(* Logix 5000 AddOnInstructionDefinition export Banner_K50Z_PD_v4; software revision 33.00 *)

TYPE Banner_K50Z_PD0_v4 :   // Process Data 0 for a K50Z.
STRUCT
   C1_Output_State : SINT;   // 0 = Inactive, 1 = Active
   C2_Output_State : SINT;   // 0 = Inactive, 1 = Active
   Stability_Z1 : SINT;   // 0 = No target or Marginal, 1 = Stable
   Stability_Z2 : SINT;   // 0 = No target or Marginal, 1 = Stable
   Measurement_1 : DINT;   // Default setting is Measurement Value for Zone 1. See IODD for all options.
   Measurement_2 : DINT;   // Default setting is Measurement Value for Zone 2. See IODD for all options.
END_STRUCT
END_TYPE

TYPE Banner_K50Z_PD1_v4 :   // Process Data 1 for a K50Z.
STRUCT
   Measurement_1 : DINT;   // Default setting is Measurement Value for Zone 1. See IODD for all options.
   Measurement_2 : DINT;   // Default setting is Measurement Value for Zone 2. See IODD for all options.
END_STRUCT
END_TYPE

TYPE Banner_K50Z_PD2_v4 :   // Process Data 2 for a K50Z.
STRUCT
   Measurement : DINT;   // Measurement Value
   Measure_Scale : DINT;   // Scale Factor for Measurement
   Stability : SINT;   // 0 = Inactive 1 = Active
   Channel_1 : SINT;   // 0 = Inactive 1 = Active
   Channel_2 : INT;   // 0 = Inactive 1 = Active
END_STRUCT
END_TYPE

TYPE Banner_K50Z_PDIO_v4 :   // Process Data for a K50Z.
STRUCT
   PDI_0 : Banner_K50Z_PD0_v4;   // Input Procoess Data for Configuration 0
   PDI_1 : Banner_K50Z_PD1_v4;   // Input Procoess Data for Configuration 1
   PDI_2 : Banner_K50Z_PD2_v4;   // Input Procoess Data for Configuration 2
   Emitter_Disable : SINT;   // 0 = Active 1 = Inactive
   PDI_DT : SINT[4];
END_STRUCT
END_TYPE

ADD_ON_INSTRUCTION Banner_K50Z_PD_v4   (* revision 4.1, vendor Banner Engineering *)
// Take raw process data and convert it to usable values.
VAR_IN_OUT
   PD : Banner_K50Z_PDIO_v4; {required}   // Process Data for a Q5X.
END_VAR
VAR_INPUT
   Configuration : SINT; {required}
   Byte_Swap : BOOL; {required}
END_VAR
VAR
   TempI : SINT[4]; {access None}
END_VAR

ROUTINE Logic   (* ladder *)
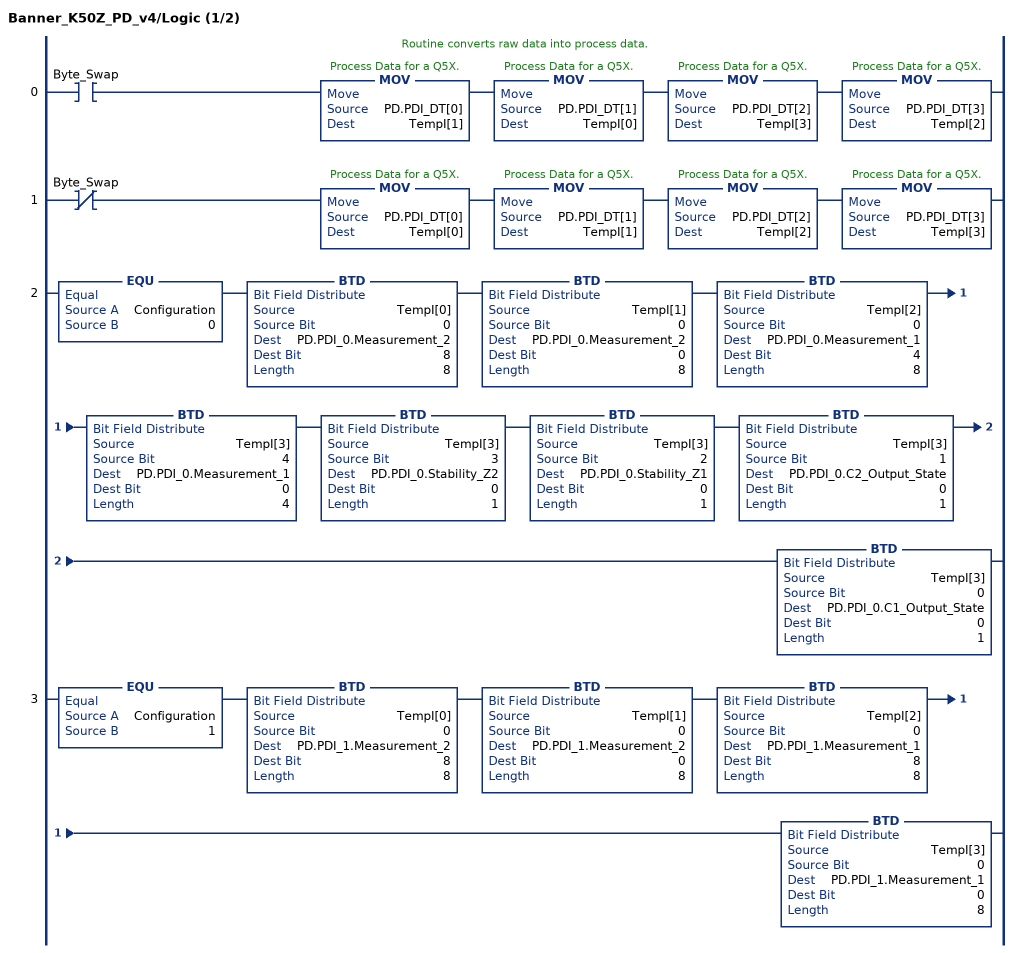
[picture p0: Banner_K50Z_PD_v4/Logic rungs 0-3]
   // Routine converts raw data into process data.
   0: XIC(Byte_Swap)MOV(PD.PDI_DT[0],TempI[1])MOV(PD.PDI_DT[1],TempI[0])MOV(PD.PDI_DT[2],TempI[3])MOV(PD.PDI_DT[3],TempI[2]);
   1: XIO(Byte_Swap)MOV(PD.PDI_DT[0],TempI[0])MOV(PD.PDI_DT[1],TempI[1])MOV(PD.PDI_DT[2],TempI[2])MOV(PD.PDI_DT[3],TempI[3]);
   2: EQU(Configuration,0)BTD(TempI[0],0,PD.PDI_0.Measurement_2,8,8)BTD(TempI[1],0,PD.PDI_0.Measurement_2,0,8)BTD(TempI[2],0,PD.PDI_0.Measurement_1,4,8)BTD(TempI[3],4,PD.PDI_0.Measurement_1,0,4)BTD(TempI[3],3,PD.PDI_0.Stability_Z2,0,1)BTD(TempI[3],2,PD.PDI_0.Stability_Z1,0,1)BTD(TempI[3],1,PD.PDI_0.C2_Output_State,0,1)BTD(TempI[3],0,PD.PDI_0.C1_Output_State,0,1);
   3: EQU(Configuration,1)BTD(TempI[0],0,PD.PDI_1.Measurement_2,8,8)BTD(TempI[1],0,PD.PDI_1.Measurement_2,0,8)BTD(TempI[2],0,PD.PDI_1.Measurement_1,8,8)BTD(TempI[3],0,PD.PDI_1.Measurement_1,0,8);
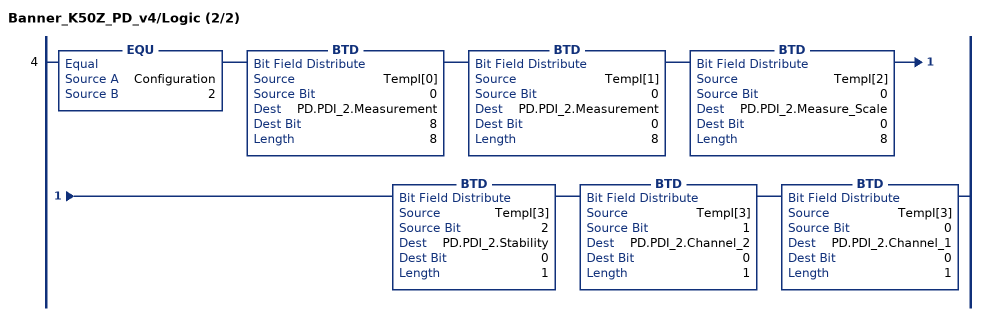
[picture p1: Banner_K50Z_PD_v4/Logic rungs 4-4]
   4: EQU(Configuration,2)BTD(TempI[0],0,PD.PDI_2.Measurement,8,8)BTD(TempI[1],0,PD.PDI_2.Measurement,0,8)BTD(TempI[2],0,PD.PDI_2.Measure_Scale,0,8)BTD(TempI[3],2,PD.PDI_2.Stability,0,1)BTD(TempI[3],1,PD.PDI_2.Channel_2,0,1)BTD(TempI[3],0,PD.PDI_2.Channel_1,0,1);
END_ROUTINE
END_ADD_ON_INSTRUCTION
